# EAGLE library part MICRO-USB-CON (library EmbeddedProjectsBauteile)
RS Components Micro USB Stecker für SONY Handy
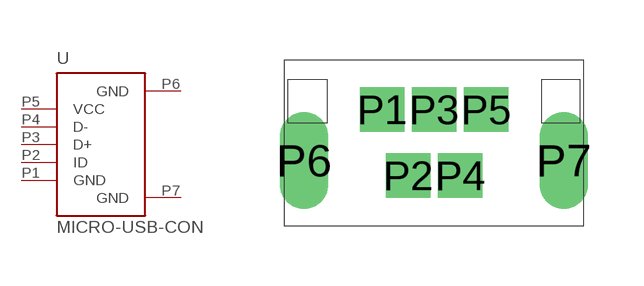
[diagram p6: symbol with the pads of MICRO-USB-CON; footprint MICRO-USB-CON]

Designator prefix -

## MICRO-USB-CON  [MICRO-USB-CON]
P1  GND
P2  ID
P3  D+
P4  D-
P5  VCC
P6  GND  pwr
P7  GND  pwr

## Footprint MICRO-USB-CON (pad centres in mm)
drill 0.6 pad 0.61 square: P1 -1.29,0.805; P2 -0.64,-0.845; P3 0.01,0.805; P4 0.66,-0.845; P5 1.31,0.805
drill 0.7 pad 0.813 long: P6 -3.24,-0.47; P7 3.26,-0.47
